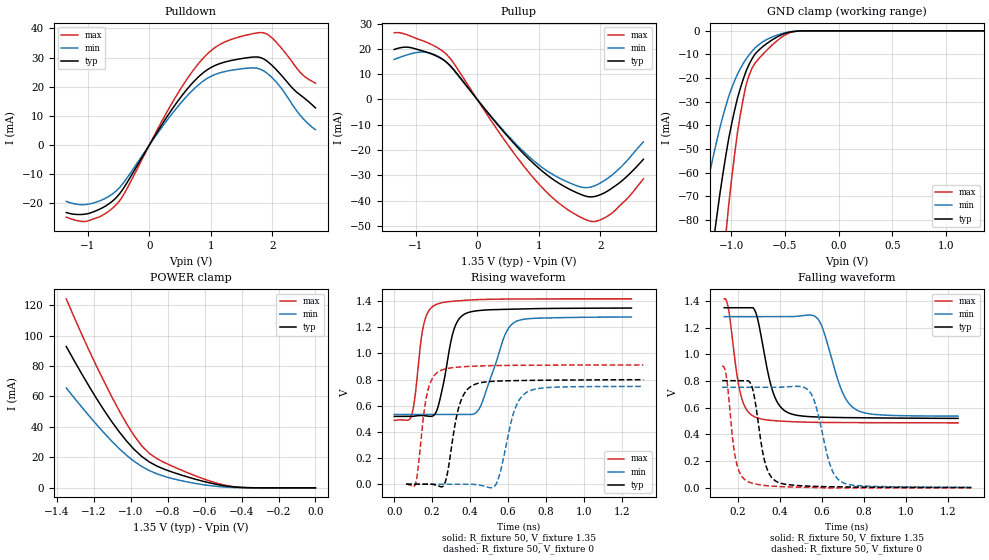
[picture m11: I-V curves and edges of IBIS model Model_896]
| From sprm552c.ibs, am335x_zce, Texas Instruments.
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| Model based on original model for BCSHTLTCSCDDVPBFZ_SSDHV
|   Sub model SR00_11MA_PADN_5PER_1P35
[model]   Model_896
|[Description]  [1.35V-3-STATE-NOTERM-SR00:11MA, IND, 5%]
|   Fastest slew rate (SR[1:0] = "00"), 0.73 * RExt = 1.325 * Iout
|   (I[2:0] = "110"), 11mA nominal with Rext = 50R,ODT off (ODT[1:0]
|   = "00") CMOS mode,Industrial temperature range (-40C to 125C,
|   25C nominal),5% power supply tolerance
|[Input Load]   NOTERM
|[Output Drive] SR00:11MA
|Voltage   1.35V
|Mode   3-STATE
Model_type   3-state
Polarity   Non-Inverting
Enable   Active-Low
Cref =  15pF
Rref =  100.0000M
Vref =  0V
Vmeas =  0.675
C_comp   1.865048p   1.679967p   1.989968p
[Temperature Range]   25   125   -40
[Voltage Range]   1.35   1.2825   1.4175
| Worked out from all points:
|   slope of the pulldown table from 0 to 0.203 V, typ, clamps not added: 29.1 ohm
|   slope of the pullup table from 0 to 0.203 V, typ, clamps not added: 32.8 ohm
|   GND clamp passes 1 mA (typ) near -0.49 V on its own axis
|   POWER clamp passes 1 mA (typ) near -0.47 V on its own axis
|   rising waveform, R_fixture 50, V_fixture 1.35: 20-80 % time 67.7ps typ, 103ps min, 47.2ps max; typ from 0.518 V to 1.35 V
|   rising waveform, R_fixture 50, V_fixture 0: 20-80 % time 62.3ps typ, 74ps min, 49.2ps max; typ from 0 V to 0.799 V
|   falling waveform, R_fixture 50, V_fixture 1.35: 20-80 % time 69.4ps typ, 90.4ps min, 52.7ps max; typ from 1.35 V to 0.521 V
|   falling waveform, R_fixture 50, V_fixture 0: 20-80 % time 51.5ps typ, 69.6ps min, 40.8ps max; typ from 0.804 V to 0.003 V
[POWER_clamp]
-1.35V    92.75mA    65.58mA    124.1mA
-1.227V   66.81mA    47.37mA    90.43mA
-1.145V   50.92mA    36.04mA    69.8mA
-1.064V   36.83mA    25.8mA     50.7mA
-981.8mV  25.17mA    17.34mA    34.14mA
-940.9mV  20.58mA    14.01mA    27.56mA
-900mV    17mA       11.33mA    22.64mA
-859.1mV  14.3mA     9.214mA    19.2mA
-736.4mV  8.769mA    4.942mA    12.14mA
-490.9mV  1.299mA    528.4uA    1.73mA
-368.2mV  117.2uA    50.88uA    117.5uA
0V        1.028nA    11.95nA    1.029nA
[Pulldown]
-1.35V    -23.15mA   -19.32mA   -24.75mA
-1.023V   -23.64mA   -20.36mA   -26.16mA
-777.3mV  -21.69mA   -18.89mA   -24.29mA
-531.8mV  -17.89mA   -15.6mA    -20.33mA
531.8mV   17.01mA    14.93mA    20.05mA
859.1mV   24.52mA    21.69mA    29.43mA
1.145V    27.94mA    24.77mA    34.48mA
1.677V    30.17mA    26.47mA    38.18mA
1.882V    29.25mA    25.13mA    38.35mA
2.086V    25.33mA    21.05mA    34.75mA
2.495V    16.49mA    9.165mA    24.02mA
2.7V      12.74mA    5.257mA    21.21mA
[Pullup]
-1.35V    19.75mA    15.81mA    26.32mA
-1.145V   20.68mA    17.58mA    25.6mA
-900mV    19.27mA    18.75mA    23.32mA
-572.7mV  15.97mA    16.13mA    19.29mA
-409.1mV  12.56mA    12.35mA    15.23mA
777.3mV   -21.99mA   -21.12mA   -26.94mA
1.186V    -30.76mA   -29mA      -37.96mA
1.555V    -36.1mA    -33.46mA   -44.78mA
1.841V    -38.46mA   -34.59mA   -48.08mA
2.045V    -37.11mA   -32.31mA   -47.03mA
2.414V    -30.78mA   -24.72mA   -39.71mA
2.7V      -23.61mA   -16.77mA   -31.32mA
[GND_clamp]
-1.35V    -159.1mA   -94.77mA   -266.2mA
-1.295V   -137.7mA   -81.77mA   -230.9mA
-1.159V   -87.19mA   -51.56mA   -145.9mA
-1.132V   -77.89mA   -46.14mA   -129.9mA
-1.05V    -52.83mA   -31.84mA   -86.44mA
-1.023V   -45.55mA   -27.75mA   -73.68mA
-940.9mV  -28.44mA   -18.28mA   -42.92mA
-859.1mV  -16.79mA   -11.75mA   -22.47mA
-804.5mV  -11.72mA   -8.559mA   -15.69mA
-722.7mV  -7.324mA   -5.162mA   -10.76mA
-395.5mV  -159.1uA   -161.1uA   -232.3uA
1.35V     1.028nA    30.09nA    754.3pA
[Ramp]
dV/dt_f 0.50696228/70.58214p  0.45733173/92.479676p 0.56509508/52.969193p
dV/dt_r 0.49402304/63.710924p 0.46813493/76.733462p 0.55815487/49.588658p
R_load = 50
[Rising Waveform]
R_fixture = 50
V_fixture = 1.35
V_fixture_min = 1.2825
V_fixture_max = 1.4175
0s        518.3mV    533.2mV    487.9mV
89.54ps   518.3mV    533.2mV    517.7mV
154.3ps   524.5mV    533.2mV    1.214V
216.7ps   540.5mV    533.2mV    1.371V
311.4ps   1.167V     533.2mV    1.399V
372.7ps   1.303V     533.2mV    1.406V
450.2ps   1.329V     582.8mV    1.412V
580.4ps   1.337V     1.131V     1.416V
637.7ps   1.339V     1.242V     1.417V
1.25ns    1.347V     1.279V     1.418V
[Rising Waveform]
R_fixture = 50
V_fixture = 0
V_fixture_min = 0
V_fixture_max = 0
62.9ps    0V         0V         0V
112.8ps   0V         0V         5.02mV
172.2ps   0V         0V         684.9mV
240.3ps   -17.09mV   0V         866.3mV
344.2ps   607.8mV    0V         896.6mV
413.9ps   756.3mV    0V         902.6mV
536.8ps   788.2mV    0V         907.7mV
632.3ps   792.1mV    559.3mV    909mV
701.1ps   793.7mV    705.4mV    909.5mV
1.313ns   799.4mV    748mV      912.1mV
[Falling Waveform]
R_fixture = 50
V_fixture = 1.35
V_fixture_min = 1.2825
V_fixture_max = 1.4175
134.9ps   1.35V      1.283V     1.417V
156ps     1.35V      1.283V     1.338V
212.3ps   1.35V      1.283V     707.6mV
273.8ps   1.348V     1.283V     537.1mV
365.4ps   727.3mV    1.283V     504.4mV
436.1ps   566.1mV    1.283V     497.6mV
582.8ps   530.8mV    1.263V     490.7mV
693.8ps   526.9mV    734.7mV    489.3mV
761.5ps   525.8mV    588.2mV    488.8mV
1.25ns    520.9mV    537.7mV    487mV
[Falling Waveform]
R_fixture = 50
V_fixture = 0
V_fixture_min = 0
V_fixture_max = 0
124.9ps   803.7mV    753.7mV    911.3mV
146.4ps   803.7mV    753.7mV    821.9mV
191.4ps   803.7mV    753.7mV    200.6mV
248.7ps   803.7mV    753.7mV    46.25mV
332.2ps   174.4mV    753.7mV    17.09mV
388.1ps   44.25mV    753.7mV    10.68mV
544.9ps   11.99mV    715.9mV    3.087mV
640.2ps   8.331mV    169.1mV    0V
698.8ps   7.112mV    40.42mV    0V
1.313ns   2.568mV    3.461mV    0V
